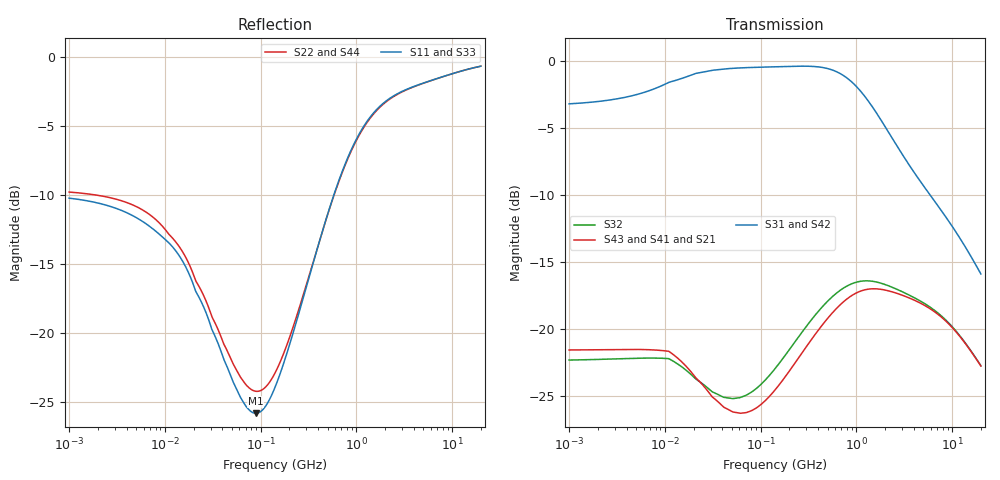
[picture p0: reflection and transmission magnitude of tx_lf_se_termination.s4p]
! Created Wed Jul 29 12:31:17 2015
# hz S db R 50
! 4 Port Network Data from SP1.SP block
! freq  dbS11  angS11  dbS12  angS12  dbS13  angS13  dbS14  angS14
!  dbS21  angS21  dbS22  angS22  dbS23  angS23  dbS24  angS24
!  dbS31  angS31  dbS32  angS32  dbS33  angS33  dbS34  angS34
!  dbS41  angS41  dbS42  angS42  dbS43  angS43  dbS44  angS44
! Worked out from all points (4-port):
!   861 points, 1 MHz to 20 GHz, reference 50 ohm
!   strongest paths, dB at 1 MHz, 11.89 MHz, 141.4 MHz, 1.682 GHz, 20 GHz:
!     S31: -3.2, -1.5, -0.4, -4.0, -15.9
!     S42: -3.4, -1.7, -0.5, -4.1, -15.9
!     S43: -21.6, -21.8, -24.5, -17.0, -22.7
!     S41: -21.6, -21.8, -24.5, -17.0, -22.7
!     S21: -21.6, -21.8, -24.5, -17.0, -22.7
!     S32: -22.3, -22.3, -23.0, -16.5, -22.7
!   lowest |S11| = -25.8 dB at 89.22 MHz (marker M1), VSWR 1.11, Z = 45.2 - j0.623 ohm
!   |S11| at or under -10 dB: start of sweep to 582.2 MHz
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1000000  -10.23 175.2  -22.31 -3.3  -3.18 2.1  -22.31 -3.3
         -21.55 -2.7  -9.79 175.5  -21.55 -2.7  -3.38 2.2
         -3.18 2.1  -22.31 -3.3  -10.23 175.2  -22.31 -3.3
         -21.55 -2.7  -3.38 2.2  -21.55 -2.7  -9.79 175.5
1.189207e7  -13.72 144.5  -22.34 -53.0  -1.51 8.2  -22.34 -53.0
            -21.83 -47.4  -13.09 146.2  -21.83 -47.4  -1.67 8.6
            -1.51 8.2  -22.34 -53.0  -13.72 144.5  -22.34 -53.0
            -21.83 -47.4  -1.67 8.6  -21.83 -47.4  -13.09 146.2
8.9221e7  -25.82 -172.3  -24.46 -137.2  -0.45 -0.4  -24.46 -137.2
          -25.90 -131.2  -24.23 -174.8  -25.90 -131.2  -0.55 -0.3
          -0.45 -0.4  -24.46 -137.2  -25.82 -172.3  -24.46 -137.2
          -25.90 -131.2  -0.55 -0.3  -25.90 -131.2  -24.23 -174.8
4.577593e8  -12.29 -109.7  -18.20 153.9  -0.48 -14.0  -18.20 153.9
            -19.54 151.5  -12.30 -112.9  -19.54 151.5  -0.60 -13.9
            -0.48 -14.0  -18.20 153.9  -12.29 -109.7  -18.20 153.9
            -19.54 151.5  -0.60 -13.9  -19.54 151.5  -12.30 -112.9
1.218257e9  -4.93 -132.9  -16.39 76.2  -2.59 -34.1  -16.39 76.2
            -17.07 72.6  -5.02 -133.7  -17.07 72.6  -2.68 -33.5
            -2.59 -34.1  -16.39 76.2  -4.93 -132.9  -16.39 76.2
            -17.07 72.6  -2.68 -33.5  -17.07 72.6  -5.02 -133.7
3.279759e9  -2.37 -156.4  -17.33 15.5  -7.35 -45.2  -17.33 15.5
            -17.56 14.2  -2.40 -156.5  -17.56 14.2  -7.34 -44.8
            -7.35 -45.2  -17.33 15.5  -2.37 -156.4  -17.33 15.5
            -17.56 14.2  -7.34 -44.8  -17.56 14.2  -2.40 -156.5
2e10  -0.67 -171.5  -22.73 -40.6  -15.88 -58.5  -22.73 -40.6
      -22.75 -40.6  -0.67 -171.5  -22.75 -40.6  -15.88 -58.5
      -15.88 -58.5  -22.73 -40.6  -0.67 -171.5  -22.73 -40.6
      -22.75 -40.6  -15.88 -58.5  -22.75 -40.6  -0.67 -171.5
